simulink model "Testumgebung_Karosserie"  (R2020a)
settings: Solver=ode4  StartTime=0.0  StopTime=Simulationszeit  FixedStep=0.01  RelTol=1e-3
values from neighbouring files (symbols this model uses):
  Fahrerlenkwinkel_value = 1.3    [Single_Testskript_Karosserie.m]    (also in Testskript_Karosserie.m = (b-a).*rand(1,1) + a)
  Gierrate_value = 2    [Single_Testskript_Karosserie.m]    (also in Testskript_Karosserie.m = (b-a).*rand(1,1) + a; Single_TestSkript_Hinterachse.m; Testskript_Hinterachse.m = (b-a).*rand(1,1) + a; Single_Testskript_Vorderachse.m)
  Jzz = 1    [Single_Testskript_Karosserie.m]    (also in Testskript_Karosserie.m = (b-a).*rand(1,1) + a)
  Laengsgeschwindigkeit_value = 8.33    [Single_Testskript_Karosserie.m]    (also in Testskript_Karosserie.m = (b-a).*rand(1,1) + a; Single_TestSkript_Hinterachse.m; Testskript_Hinterachse.m = (b-a).*rand(1,1) + a)
  lh = 1.3    [Single_Testskript_Karosserie.m]    (also in Testskript_Karosserie.m = (b-a).*rand(1,1) + a; Single_TestSkript_Hinterachse.m; Testskript_Hinterachse.m = (b-a).*rand(1,1) + a)
  lv = 1.3    [Single_Testskript_Karosserie.m]    (also in Testskript_Karosserie.m = (b-a).*rand(1,1) + a; Single_Testskript_Vorderachse.m = 1.5; Testskript_Vorderachse.m = (b-a).*rand(1,1) + a)
  m = 1500    [Single_Testskript_Karosserie.m]    (also in Testskript_Karosserie.m = (b-a).*rand(1,1) + a)
  Querbeschleunigung_value = 3    [Single_Testskript_Karosserie.m]    (also in Testskript_Karosserie.m = (b-a).*rand(1,1) + a; Testskript_Ausgabe.m = (b-a).*rand(1,1) + a)
  Seitenfuerungskraft_K_h_value = 100000    [Single_Testskript_Karosserie.m]    (also in Testskript_Karosserie.m = (b-a).*rand(1,1) + a)
  Seitenfuerungskraft_K_v_value = 80000    [Single_Testskript_Karosserie.m]    (also in Testskript_Karosserie.m = (b-a).*rand(1,1) + a)
  Seitenfuerungskraft_R_h_value = 100000    [Single_Testskript_Karosserie.m]    (also in Testskript_Karosserie.m = (b-a).*rand(1,1) + a)
  Seitenfuerungskraft_R_v_value = 80000    [Single_Testskript_Karosserie.m]    (also in Testskript_Karosserie.m = (b-a).*rand(1,1) + a)

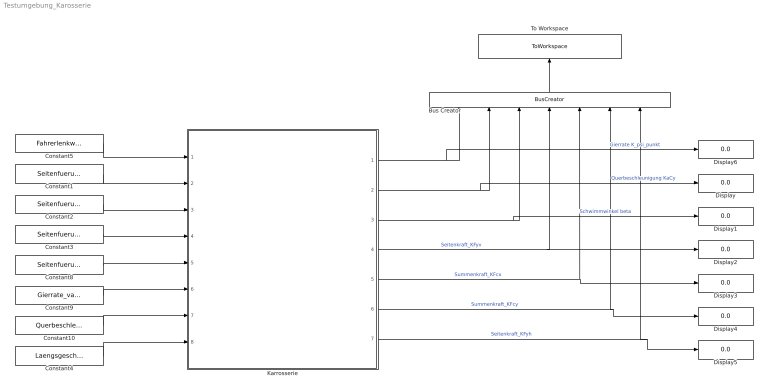
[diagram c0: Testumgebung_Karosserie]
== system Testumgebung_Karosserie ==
  Bus Creator : BusCreator  Inputs=7
  Constant1 : Constant  Value=Seitenfuerungskraft_K_v_value
  Constant10 : Constant  Value=Querbeschleunigung_value
  Constant2 : Constant  Value=Seitenfuerungskraft_K_h_value
  Constant3 : Constant  Value=Seitenfuerungskraft_R_v_value
  Constant4 : Constant  Value=Laengsgeschwindigkeit_value
  Constant5 : Constant  Value=Fahrerlenkwinkel_value
  Constant8 : Constant  Value=Seitenfuerungskraft_R_h_value
  Constant9 : Constant  Value=Gierrate_value
  Display{,1..6} (7 alike) : Display
  Karrosserie : Subsystem
  To Workspace : ToWorkspace  VariableName=simout  SaveFormat=Timeseries  SampleTime=-1
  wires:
  Constant5/1 -> Karrosserie/1(Fahrerlenkwinkel teta_v)
  Constant1/1 -> Karrosserie/2(Seitenführungskraft Vorderachse KFyv)
  Constant2/1 -> Karrosserie/3(Seitenführungskraft Hinterachse KFyh)
  Constant3/1 -> Karrosserie/4(Seitenführungskraft vorderachse RFyv)
  Constant8/1 -> Karrosserie/5(Seitenführungskraft hintererachse RFyh)
  Constant9/1 -> Karrosserie/6(Gierrate K_psi_punkt)
  Constant10/1 -> Karrosserie/7(Querbeschleunigung KaCy)
  Constant4/1 -> Karrosserie/8(Fahrzeuglängsgeschwindigkeit KvCx)
  Bus Creator/1 -> To Workspace/1
  Karrosserie/4(Seitenführungskraft vorderachse KFyv) -> Display2/1, Bus Creator/4  "Seitenkraft_KFyv"
  Karrosserie/5(Summenkraft KFcx) -> Display3/1, Bus Creator/5  "Summenkraft_KFcx"
  Karrosserie/6(Summenkraft KFcy) -> Display4/1, Bus Creator/6  "Summenkraft_KFcy"
  Karrosserie/7(Seitenführungskraft hinterachse KFyh) -> Bus Creator/7, Display5/1  "Seitenkraft_KFyh"
  Karrosserie/1(Gierrate k_psi_punkt) -> Display6/1, Bus Creator/1  "Gierrate K_psi_punkt"
  Karrosserie/2(Querbeschleunigung kAcY) -> Display/1, Bus Creator/2  "Querbeschleunigung KaCy"
  Karrosserie/3(Schwimmwinkel beta) -> Display1/1, Bus Creator/3  "Schwimmwinkel beta"

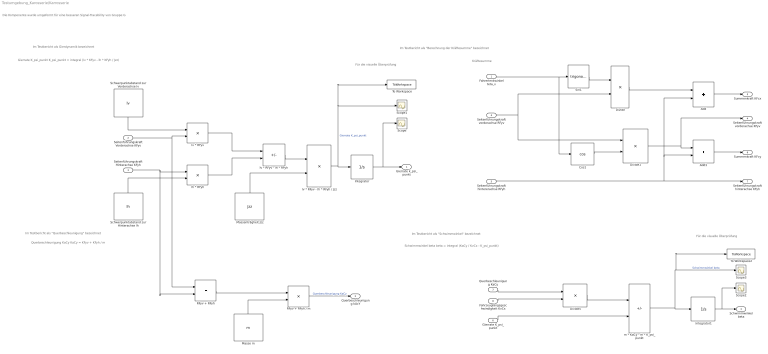
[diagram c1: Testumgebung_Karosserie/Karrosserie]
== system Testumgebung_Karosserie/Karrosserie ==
  note: Für die visuelle Überprüfung
  note: Die Komponente wurde umgeformt für eine besseren Signal-Tracebility von Gruppe G
  note: Im Testbericht als "Schwimmwinkel" bezeichnet
  note: Im Testbericht als "Berechnung der Kräftesumme" bezeichnet
  note: Im Testbericht als "Querbeschleunigung" bezeichnet
  note: Im Testbericht als Gierdynamik bezeichnet
  note: Kräftesumme
  note: Gierrate K_psi_punkt K_psi_punkt = integral (lv * KFyv - lh * KFyh / Jzz)
  note: Querbeschleunigung KaCy KaCy = KFyv + KFyh / m
  note: Schwimmwinkel beta beta = integral (KaCy / KvCx - K_psi_punkt)
  note: Für die visuelle Überprüfung
  Fahrerlenkwinkel teta_v : Inport
  Seitenführungskraft Vorderachse KFyv : Inport  Port=2
  Seitenführungskraft Hinterachse KFyh : Inport  Port=3
  Seitenführungskraft vorderachse RFyv : Inport  Port=4
  Seitenführungskraft hintererachse RFyh : Inport  Port=5
  Gierrate K_psi_punkt : Inport  Port=6
  Querbeschleunigung KaCy : Inport  Port=7
  Fahrzeuglängsgeschwindigkeit KvCx : Inport  Port=8
  Add : Sum
  Add1 : Sum
  Cos1 : Trigonometry  Operator=cos
  Divide : Product
  Divide1 : Product
  Divide5 : Product  Inputs=*/
  Integrator : Integrator
  Integrator1 : Integrator
  Masse m : Constant  Value=m
  Massenträgheit Jzz : Constant  Value=Jzz
  RFyv + RFyh : Sum
  RFyv + RFyh / m : Product  Inputs=*/
  Schwerpunktabstand zur Hinterachse lh : Constant  Value=lh
  Schwerpunktabstand zur Vorderachse lv : Constant  Value=lv
  Scope{,1..3} (4 alike) : Scope
  Sin1 : Trigonometry
  To Workspace : ToWorkspace  VariableName=Psipp  SaveFormat=Timeseries  SampleTime=-1
  To Workspace2 : ToWorkspace  VariableName=betap  SaveFormat=Timeseries  SampleTime=-1
  lh * RFyh : Product
  lv * RFyv : Product
  lv * RFyv - lh * RFyh : Sum  Inputs=+-
  lv * RFyv - lh * RFyh / Jzz : Product  Inputs=*/
  m * KaCy - m * K_psi_punkt : Sum  Inputs=+-
  Gierrate k_psi_punkt : Outport
  Querbeschleunigung kAcY : Outport  Port=2
  Schwimmwinkel beta : Outport  Port=3
  Seitenführungskraft vorderachse KFyv : Outport  Port=4
  Summenkraft KFcx : Outport  Port=5
  Summenkraft KFcy : Outport  Port=6
  Seitenführungskraft hinterachse KFyh : Outport  Port=7
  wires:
  RFyv + RFyh / m/1 -> Querbeschleunigung kAcY/1  "Querbeschleunigung KaCy"
  m * KaCy - m * K_psi_punkt/1 -> To Workspace2/1, Scope3/1, Integrator1/1  "Schwimmwinkel beta"
  lv * RFyv - lh * RFyh/1 -> lv * RFyv - lh * RFyh / Jzz/1
  lv * RFyv/1 -> lv * RFyv - lh * RFyh/1
  Massenträgheit Jzz/1 -> lv * RFyv - lh * RFyh / Jzz/2
  lh * RFyh/1 -> lv * RFyv - lh * RFyh/2
  Schwerpunktabstand zur Vorderachse lv/1 -> lv * RFyv/1
  Schwerpunktabstand zur Hinterachse lh/1 -> lh * RFyh/2
  Masse m/1 -> RFyv + RFyh / m/2
  RFyv + RFyh/1 -> RFyv + RFyh / m/1
  Fahrerlenkwinkel teta_v/1 -> Cos1/1, Sin1/1
  Sin1/1 -> Divide/1
  Seitenführungskraft vorderachse RFyv/1 -> Divide1/1, Divide/2
  Divide/1 -> Add/1
  Seitenführungskraft hintererachse RFyh/1 -> Add/2, Add1/2, Seitenführungskraft hinterachse KFyh/1
  Add/1 -> Summenkraft KFcx/1
  Divide1/1 -> Seitenführungskraft vorderachse KFyv/1, Add1/1
  Add1/1 -> Summenkraft KFcy/1
  Seitenführungskraft Vorderachse KFyv/1 -> RFyv + RFyh/1, lv * RFyv/2
  Seitenführungskraft Hinterachse KFyh/1 -> RFyv + RFyh/2, lh * RFyh/1
  Querbeschleunigung KaCy/1 -> Divide5/1
  Fahrzeuglängsgeschwindigkeit KvCx/1 -> Divide5/2
  Divide5/1 -> m * KaCy - m * K_psi_punkt/1
  Gierrate K_psi_punkt/1 -> m * KaCy - m * K_psi_punkt/2
  lv * RFyv - lh * RFyh / Jzz/1 -> To Workspace/1, Scope1/1, Integrator/1  "Gierrate K_psi_punkt"
  Integrator/1 -> Scope/1, Gierrate k_psi_punkt/1
  Cos1/1 -> Divide1/2
  Integrator1/1 -> Scope2/1, Schwimmwinkel beta/1
